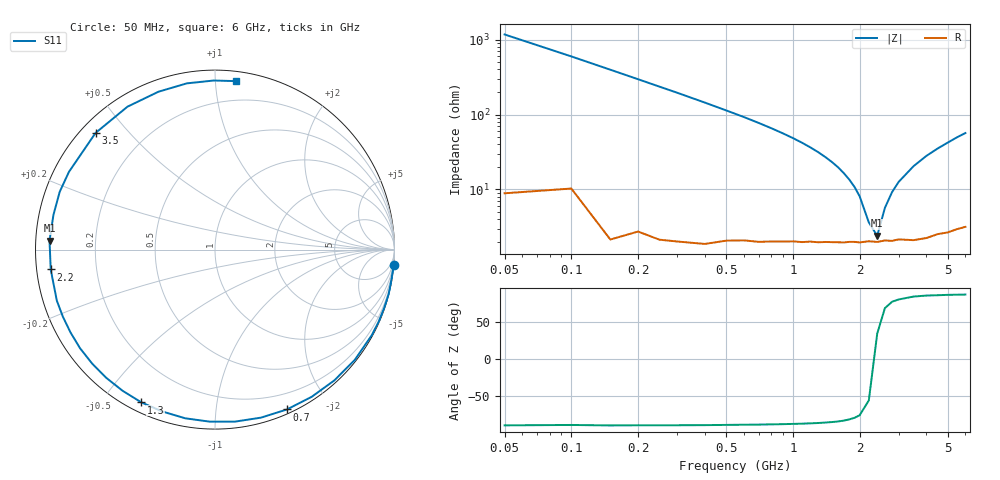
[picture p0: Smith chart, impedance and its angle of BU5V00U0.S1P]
! Infineon Technologies  Discrete & RF Semiconductors
! BB 833
! Si Tuning Diode in SOD323
! VR = 5 V
! S-Parameters:  June  1999
# GHz  S  MA  R  50
!  f  S11
! GHz  MAG  ANG
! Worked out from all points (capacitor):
!   34 points, 50 MHz to 6 GHz, reference 50 ohm
!   read as one part to ground: C = 2.67 pF near 50 MHz
!   lowest |Z| = 2.41 ohm at 2.4 GHz (marker M1)
!   series resonance near 2.338 GHz, so ESL is about 1.7 nH
!   S11 on the Smith chart (normalised r, x): 50 MHz: 0, -23; 700 MHz: 0.04, -1.55; 1.3 GHz: 0.04, -0.63; 2.2 GHz: 0.04, -0.06; 3.5 GHz: 0.04, +0.41; 6 GHz: 0.06, +1.13
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0.05  0.9993 -4.9
0.15  0.9987 -14.4
0.3  0.995 -28.7
0.4  0.992 -38.2
0.5  0.9866 -47.6
0.6  0.9813 -56.7
0.7  0.9766 -65.8
0.8  0.9707 -74.7
0.9  0.9649 -83.4
1  0.9589 -91.8
1.1  0.9544 -100.0
1.3  0.9449 -115.7
1.4  0.9401 -123.2
1.6  0.9338 -137.1
1.7  0.9313 -143.9
1.9  0.9263 -156.2
2  0.926 -162.1
2.2  0.9219 -173.1
2.4  0.9233 176.9
2.6  0.9207 167.9
2.8  0.9232 159.6
3  0.9219 152.0
3.5  0.9302 135.7
4  0.9338 121.5
4.5  0.9343 109.7
5  0.9394 99.6
5.5  0.9421 90.4
6  0.9459 82.9
